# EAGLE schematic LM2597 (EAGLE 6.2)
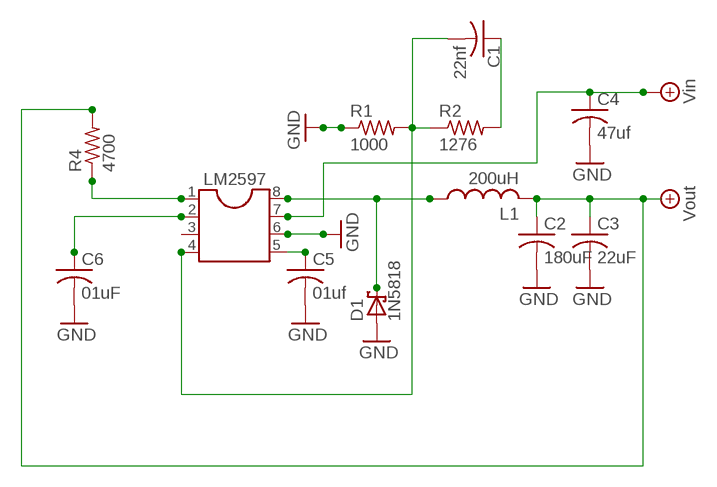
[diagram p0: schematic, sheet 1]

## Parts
C1  22nf  C-US050-025X075  [C050-025X075]
C2  180uF  C-US050-025X075  [C050-025X075]
C3  22uF  C-US050-025X075  [C050-025X075]
C4  47uf  C-US050-025X075  [C050-025X075]
C5  01uf  C-US050-025X075  [C050-025X075]
C6  01uF  C-US050-025X075  [C050-025X075]
D1  1N5818  1N5908  [C4111-15]
L1  200uH  L-USL1812  [L1812]
LM2597  DIL8  [DIL08]
R1  1000  R-US_0414/15  [0414/15]
R2  1276  R-US_0414/15  [0414/15]
R4  4700  R-US_0414/15  [0414/15]

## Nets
GND: C2.2 C3.2 C4.2 C5.2 C6.2 D1.A LM2597.6 R1.1
N$1: LM2597.1 R4.1
N$2: C6.1 LM2597.2
N$3: C1.2 LM2597.4 R1.2
N$4: D1.C L1.1 LM2597.8
N$5: C5.1 LM2597.5
N$6: C2.1 C3.1 L1.2 ; supply symbol labelled Vout
N$7: C1.1 R2.2
N$8: C4.1 LM2597.7 ; supply symbol labelled Vin
N$9: R4.2
Unconnected: LM2597.3 R2.1

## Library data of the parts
C1-C6 = resistor:C-US: CAPACITOR, American symbol
D1 = diode:1N5908: DIODE
L1 = resistor:L-US: INDUCTOR, American symbol
LM2597 = ic-package:DIL8: Dual In Line / Socket
R1 R2 R4 = resistor:R-US_: RESISTOR, American symbol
